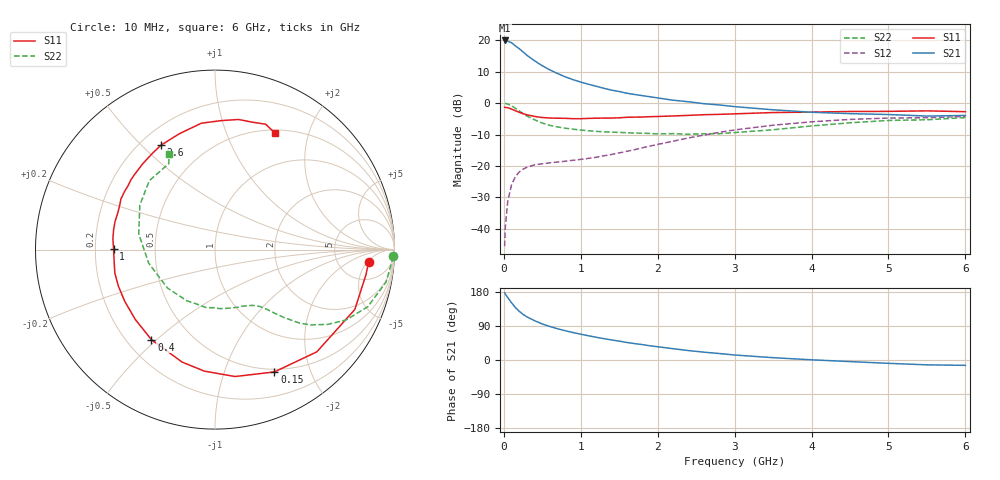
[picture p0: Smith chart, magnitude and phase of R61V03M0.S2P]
! SIEMENS Small Signal Semiconductors
! BFR193
! Si NPN RF Bipolar Junction Transistor in SOT23
! VCE = 1 V  IC = 3 mA
! Common Emitter S-Parameters:  May  1996
# GHz  S  MA  R  50
!  f  S11  S21  S12  S22
! GHz  MAG  ANG  MAG  ANG  MAG  ANG  MAG  ANG
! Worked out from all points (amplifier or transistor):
!   36 points, 10 MHz to 6 GHz, reference 50 ohm
!   highest |S21| = 19.9 dB at 10 MHz (marker M1)
!   |S21| within 3 dB of that: start of sweep to 218.8 MHz
!   unconditionally stable (mu >= 1): 1.013 GHz to 2.192 GHz
!   at 250 MHz: K = 0.31, MSG = 18.7 dB, |S12| = -21.0 dB
!   at 1.4 GHz: K = 1.12, MAG = 8.2 dB, |S12| = -16.3 dB
!   at 6 GHz: K = 1.00, MSG = 0.1 dB, |S12| = -4.2 dB
!   S11 on the Smith chart (normalised r, x): 10 MHz: 10, -5; 150 MHz: 0.47, -1.49; 400 MHz: 0.30, -0.48; 1 GHz: 0.28, +0.00; 2.6 GHz: 0.28, +0.57; 6 GHz: 0.53, +1.50
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0.01  0.8592 -4.6  9.938 177.3  0.0053 85.1  0.9942 -2.2
0.02  0.8526 -9.5  9.75 173.9  0.011 84.5  0.9865 -4.4
0.05  0.8474 -23.2  9.679 165.0  0.0269 77.8  0.9699 -10.8
0.1  0.804 -45.1  9.133 151.1  0.0503 67.4  0.9088 -20.5
0.15  0.7576 -64.1  8.136 138.6  0.0676 58.0  0.8293 -28.2
0.2  0.716 -81.0  7.357 128.7  0.0804 51.5  0.753 -33.6
0.25  0.6797 -95.0  6.533 120.3  0.089 46.2  0.6802 -38.1
0.3  0.6529 -106.3  5.772 113.9  0.0956 42.8  0.624 -41.0
0.4  0.6141 -125.2  4.713 103.6  0.1044 38.4  0.5427 -44.4
0.5  0.5906 -138.8  3.93 95.1  0.1085 36.3  0.4824 -47.0
0.6  0.5794 -150.3  3.372 88.3  0.1124 36.1  0.4426 -48.9
0.8  0.5732 -166.8  2.614 77.2  0.1193 37.4  0.3989 -52.3
1  0.5652 179.4  2.164 68.1  0.1274 41.2  0.3732 -56.4
1.1  0.572 174.0  1.998 63.9  0.1322 43.0  0.3638 -59.2
1.3  0.5785 164.2  1.723 56.4  0.1453 47.0  0.3493 -64.6
1.6  0.5953 151.6  1.435 46.2  0.1713 51.6  0.3383 -74.4
2.2  0.625 130.2  1.114 29.8  0.2477 54.0  0.3272 -98.6
2.6  0.6546 117.5  0.98 20.7  0.3103 50.9  0.3256 -118.8
3.5  0.7085 96.1  0.783 6.1  0.4452 36.6  0.377 -168.4
4.5  0.7366 79.8  0.681 -4.2  0.5507 18.5  0.4868 149.4
5.5  0.7535 68.0  0.623 -12.8  0.5851 1.5  0.5436 118.3
6  0.7312 63.0  0.637 -14.1  0.6175 -3.3  0.5893 115.7
